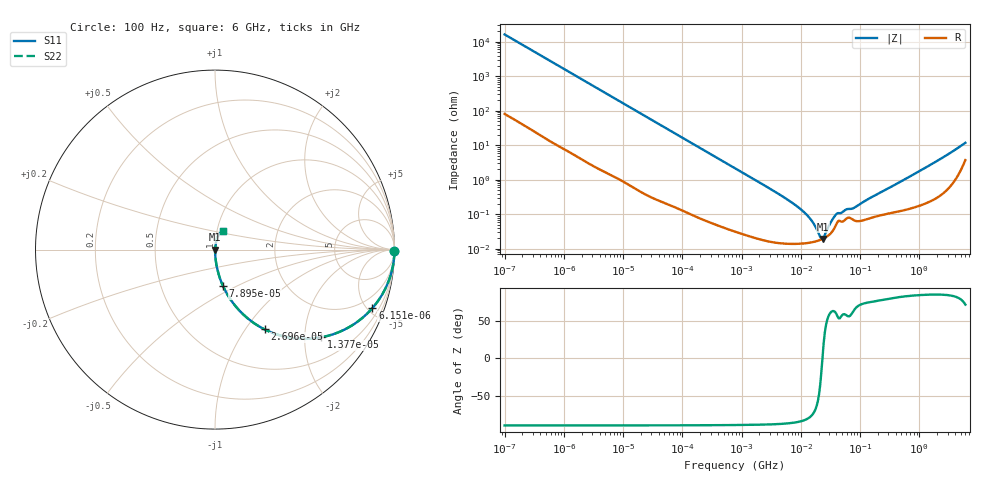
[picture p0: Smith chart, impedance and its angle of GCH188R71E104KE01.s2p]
!Murata Part Number: GCH188R71E104KE01
!These Parameters are Measured in Series Mode Connection
!Data Generated on Mar 13, 2026
!  o--ll--o
!Port1  Port2
!  o------o
!Operation Temp=25[degC], DC Bias Voltage=0[V]
!Freq. Start=100[Hz] Stop=6[GHz] 401[Steps]
# Hz S RI R 50
!Freq.(Hz) S11(Real) S11(Imag) S21(Real) S21(Imag) S12(Real) S12(Imag) S22(Real) S22(Imag)
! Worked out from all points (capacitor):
!   401 points, 100 Hz to 6 GHz, reference 50 ohm
!   read as one part in series: C = 97.4 nF near 109 Hz
!   lowest |Z| = 19.3 mohm at 23.28 MHz (marker M1)
!   series resonance near 23.16 MHz, so ESL is about 480 pH
!   S11 on the Smith chart (normalised r, x): 100 Hz: open; 6.151 kHz: 1.03, -5.37; 13.77 kHz: 1.01, -2.41; 26.96 kHz: 1.01, -1.23; 78.95 kHz: 1.00, -0.42; 6 GHz: 1.07, +0.22
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100  0.9999 -0.00613  6.81e-05 0.00613  6.81e-05 0.00613  0.9999 -0.00613
627  0.9984 -0.0381  0.00164 0.0381  0.00164 0.0381  0.9984 -0.0381
2008  0.9848 -0.1201  0.0152 0.1201  0.0152 0.1201  0.9848 -0.1201
6151  0.8769 -0.326  0.1231 0.326  0.1231 0.326  0.8769 -0.326
13772  0.5908 -0.489  0.4092 0.489  0.4092 0.489  0.5908 -0.489
26957  0.276 -0.4443  0.724 0.4443  0.724 0.4443  0.276 -0.4443
40335  0.1466 -0.3507  0.8534 0.3507  0.8534 0.3507  0.1466 -0.3507
78952  0.044 -0.2014  0.956 0.2014  0.956 0.2014  0.044 -0.2014
211427  0.00694 -0.0786  0.9931 0.0786  0.9931 0.0786  0.00694 -0.0786
774597  0.000787 -0.0217  0.9992 0.0217  0.9992 0.0217  0.000787 -0.0217
6948629  0.000144 -0.00223  0.9999 0.00223  0.9999 0.00223  0.000144 -0.00223
1.137099e7  0.000145 -0.00114  0.9999 0.00114  0.9999 0.00114  0.000145 -0.00114
1.555665e7  0.000156 -0.000607  0.9998 0.000607  0.9998 0.000607  0.000156 -0.000607
2.128304e7  0.000181 -0.000127  0.9998 0.000127  0.9998 0.000127  0.000181 -0.000127
2.327686e7  0.000193 7.7e-06  0.9998 -7.7e-06  0.9998 -7.7e-06  0.000193 7.7e-06
2.545746e7  0.000209 0.000144  0.9998 -0.000144  0.9998 -0.000144  0.000209 0.000144
3.330331e7  0.000305 0.000585  0.9997 -0.000585  0.9997 -0.000585  0.000305 0.000585
3.983537e7  0.000522 0.000875  0.9995 -0.000875  0.9995 -0.000875  0.000522 0.000875
5.960426e7  0.000766 0.00118  0.9992 -0.00118  0.9992 -0.00118  0.000766 0.00118
7.797396e7  0.000681 0.00136  0.9993 -0.00136  0.9993 -0.00136  0.000681 0.00136
3.124326e8  0.0011 0.00578  0.9989 -0.00578  0.9989 -0.00578  0.0011 0.00578
6e9  0.0472 0.1032  0.9528 -0.1032  0.9528 -0.1032  0.0472 0.1032
